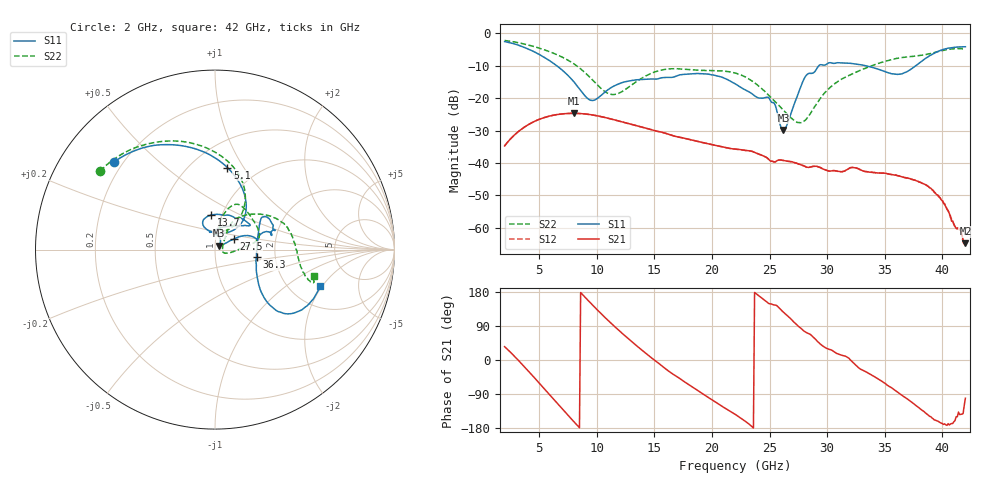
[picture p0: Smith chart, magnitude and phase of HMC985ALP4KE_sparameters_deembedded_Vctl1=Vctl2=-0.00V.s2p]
!s2p File: Measurements: S11, S21, S12, S22
# GHz S dB R 50.0
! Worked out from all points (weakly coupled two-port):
!   401 points, 2 GHz to 42 GHz, reference 50 ohm
!   highest |S21| = -24.69 dB at 8 GHz (marker M1); lowest = -64.8 dB at 42 GHz (marker M2)
!   lowest |S11| = -29.8 dB at 26.2 GHz (marker M3), VSWR 1.07, Z = 52.5 + j2.21 ohm
!   |S11| at or under -10 dB: 6.525 GHz to 29.28 GHz (22.75 GHz wide, 127 % of centre); 33.34 GHz to 37.7 GHz (4.358 GHz wide, 12.3 % of centre)
!   |S22| runs from -27.6 to -2.2 dB; largest |S21 - S12| = 0.00014
!   S11 on the Smith chart (normalised r, x): 2 GHz: 0.16, +0.36; 5.1 GHz: 0.73, +0.85; 13.7 GHz: 0.89, +0.35; 27.5 GHz: 1.22, +0.15; 36.3 GHz: 1.59, -0.14; 42 GHz: 2.89, -1.91
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2  -2.54 139.3  -34.75 35.2  -34.74 35.3  -2.21 145.7
3.5  -4.06 111.3  -29.48 -10.7  -29.49 -10.7  -3.15 122.0
5.1  -6.71 81.3  -26.41 -64.1  -26.42 -64.2  -4.68 97.7
8  -14.92 44.7  -24.69 -162.4  -24.70 -162.4  -9.40 60.1
8.7  -18.10 51.4  -24.80 174.7  -24.80 174.7  -11.28 54.6
9.7  -20.70 87.4  -25.23 143.0  -25.23 142.9  -14.63 51.8
11.3  -16.64 115.9  -26.49 95.3  -26.50 95.3  -18.86 67.9
13.7  -14.29 96.7  -28.74 31.5  -28.74 31.5  -14.31 77.2
15.4  -13.94 73.0  -30.33 -9.3  -30.33 -9.3  -11.53 68.4
19.4  -12.51 34.7  -33.88 -93.4  -33.89 -93.3  -11.47 34.2
22  -15.56 52.2  -35.72 -143.1  -35.73 -143.1  -12.25 13.0
25  -20.23 97.5  -39.18 148.3  -39.20 148.3  -19.39 -5.0
26.2  -29.84 40.8  -39.23 126.2  -39.26 126.3  -23.72 -18.3
27.5  -18.45 29.5  -40.33 89.0  -40.36 88.9  -27.51 -5.4
28.1  -13.39 20.6  -41.08 74.3  -41.10 74.1  -26.82 20.6
28.7  -12.34 12.7  -41.11 63.1  -41.11 63.1  -23.85 40.3
31  -9.09 23.3  -42.59 15.2  -42.63 15.3  -14.69 57.6
33.3  -9.96 34.4  -42.65 -30.3  -42.66 -30.4  -10.82 43.2
35.4  -12.26 12.5  -43.50 -70.2  -43.45 -69.8  -8.29 26.3
36.3  -12.58 -10.0  -44.06 -89.2  -44.05 -88.9  -7.62 18.3
39.4  -5.96 -43.8  -49.30 -158.8  -49.38 -158.4  -5.82 -14.8
42  -4.15 -19.1  -64.83 -100.9  -65.68 -102.9  -4.88 -15.0
